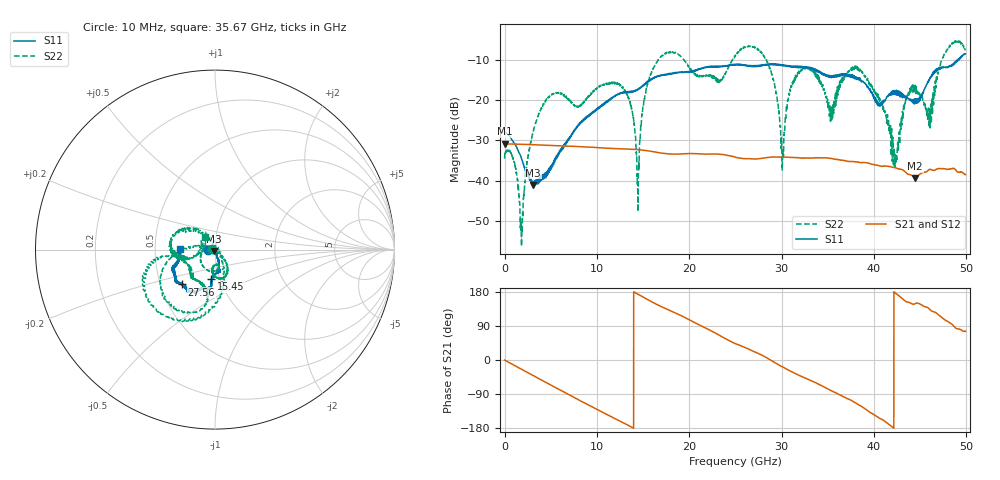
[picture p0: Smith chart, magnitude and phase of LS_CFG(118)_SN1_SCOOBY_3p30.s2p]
!Keysight Technologies,N5245B,MY58422026,A.13.80.08
!Date: Friday, March 20, 2020 00:04:15
!Correction: S11(Full 2 Port(1,2))
!S21(Full 2 Port(1,2))
!S12(Full 2 Port(1,2))
!S22(Full 2 Port(1,2))
!S2P File: Measurements: S11, S21, S12, S22:
# Hz S DB R 50.0
!freq dBS11 angS11 dBS21 angS21 dBS12 angS12 dBS22 angS22
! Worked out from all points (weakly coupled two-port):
!   4991 points, 10 MHz to 49.91 GHz, reference 50 ohm
!   highest |S21| = -30.83 dB at 50 MHz (marker M1); lowest = -39.4 dB at 44.46 GHz (marker M2)
!   lowest |S11| = -41.1 dB at 3.11 GHz (marker M3), VSWR 1.02, Z = 49.5 - j0.726 ohm
!   |S11| at or under -10 dB: start of sweep to 49.01 GHz; 49.05122 GHz to 49.10777 GHz (56.55 MHz wide, 0.115 % of centre); 49.19092 GHz to 49.20564 GHz (14.72 MHz wide, 0.0299 % of centre)
!   |S22| runs from -56.3 to -5.1 dB; largest |S21 - S12| = 0.00027
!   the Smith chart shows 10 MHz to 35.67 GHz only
!   S11 on the Smith chart (normalised r, x): 10 MHz: 0.92, -0.00; 15.45 GHz: 0.91, -0.31; 27.56 GHz: 0.65, -0.27; 35.67 GHz: 0.67, +0.00
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1e7  -28.00 -176.1  -30.84 -0.2  -30.80 -0.4  -34.55 177.1
5e7  -27.98 179.1  -30.83 -0.8  -30.83 -0.8  -33.13 -176.3
1.83e9  -34.39 -171.2  -30.96 -24.3  -30.94 -24.3  -56.22 -14.6
3.11e9  -41.09 -123.8  -31.07 -41.1  -31.06 -41.1  -27.70 159.6
8.33e9  -25.58 -72.9  -31.56 -109.3  -31.56 -109.2  -21.08 -92.5
1.276e10  -18.16 -76.2  -32.12 -164.4  -32.12 -164.3  -16.73 -62.9
1.445e10  -17.36 -88.7  -32.29 173.7  -32.29 173.8  -45.95 -107.0
1.545e10  -15.61 -96.8  -32.58 160.1  -32.57 160.2  -16.14 175.8
1.665e10  -14.04 -96.4  -33.02 144.8  -33.01 144.9  -9.97 -157.2
2.496e10  -11.19 -123.1  -34.12 43.7  -34.11 43.9  -9.07 -167.9
2.756e10  -11.46 -133.3  -34.54 16.3  -34.55 16.6  -7.73 -110.0
3.011e10  -11.42 -143.8  -34.22 -17.9  -34.23 -17.6  -34.51 16.8
3.116e10  -11.57 -148.7  -34.25 -31.6  -34.25 -31.3  -15.61 140.1
3.328e10  -12.08 -158.9  -34.37 -55.6  -34.37 -55.2  -12.35 -175.3
3.567e10  -14.16 179.5  -34.62 -84.3  -34.54 -83.7  -20.94 127.8
3.816e10  -14.81 172.2  -35.37 -115.3  -35.31 -115.5  -11.58 -174.5
4.16e10  -18.58 104.0  -36.47 -169.4  -36.50 -169.5  -25.74 67.5
4.233e10  -17.84 103.1  -36.83 176.9  -36.84 177.0  -33.65 166.0
4.446e10  -19.87 54.1  -39.38 148.6  -39.36 148.9  -16.44 -7.2
4.6e10  -15.13 9.6  -37.23 134.7  -37.24 134.8  -24.49 112.3
4.771e10  -11.77 7.3  -37.08 105.5  -37.09 105.7  -8.16 -80.0
4.991e10  -8.45 -12.6  -38.51 76.0  -38.53 76.0  -7.38 -14.6
